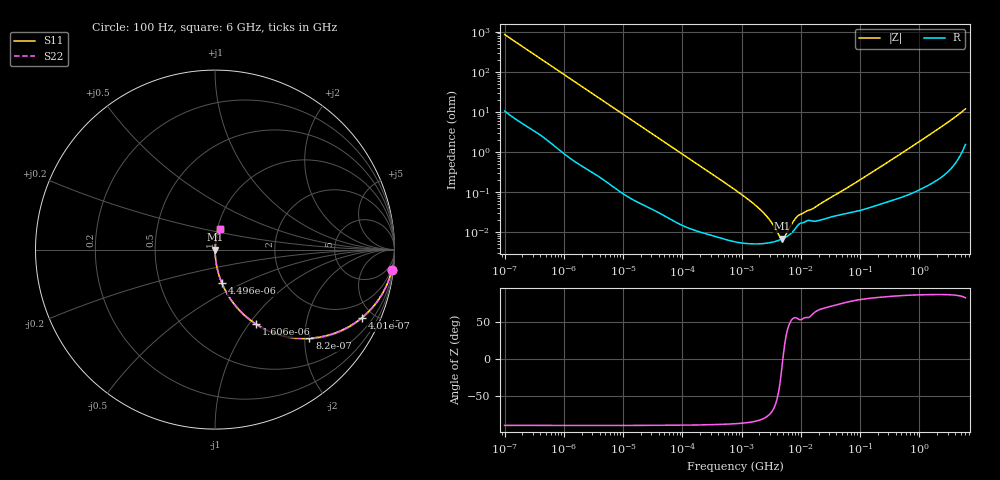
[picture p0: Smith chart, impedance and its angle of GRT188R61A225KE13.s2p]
!Murata Part Number: GRT188R61A225KE13
!These Parameters are Measured in Series Mode Connection
!Data Generated on Jun 19, 2026
!  o--ll--o
!Port1  Port2
!  o------o
!Operation Temp=25[degC], DC Bias Voltage=0[V]
!Freq. Start=100[Hz] Stop=6[GHz] 401[Steps]
# Hz S RI R 50
!Freq.(Hz) S11(Real) S11(Imag) S21(Real) S21(Imag) S12(Real) S12(Imag) S22(Real) S22(Imag)
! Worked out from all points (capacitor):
!   401 points, 100 Hz to 6 GHz, reference 50 ohm
!   read as one part in series: C = 1.87 uF near 109 Hz
!   lowest |Z| = 6.86 mohm at 4.857 MHz (marker M1)
!   series resonance near 4.978 MHz, so ESL is about 550 pH
!   S11 on the Smith chart (normalised r, x): 100 Hz: 1, -17; 401 Hz: 1.05, -4.29; 820 Hz: 1.02, -2.11; 1.606 kHz: 1.01, -1.08; 4.496 kHz: 1.00, -0.39; 6 GHz: 1.03, +0.24
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100  0.985 -0.1157  0.015 0.1157  0.015 0.1157  0.985 -0.1157
224  0.9332 -0.2437  0.0668 0.2437  0.0668 0.2437  0.9332 -0.2437
401  0.8183 -0.3795  0.1817 0.3795  0.1817 0.3795  0.8183 -0.3795
820  0.5256 -0.4939  0.4744 0.4939  0.4744 0.4939  0.5256 -0.4939
1122  0.3742 -0.4788  0.6258 0.4788  0.6258 0.4788  0.3742 -0.4788
1606  0.2281 -0.4146  0.7719 0.4146  0.7719 0.4146  0.2281 -0.4146
2008  0.16 -0.3615  0.84 0.3615  0.84 0.3615  0.16 -0.3615
4496  0.0382 -0.1864  0.9618 0.1864  0.9618 0.1864  0.0382 -0.1864
11514  0.00657 -0.0757  0.9934 0.0757  0.9934 0.0757  0.00657 -0.0757
40335  0.000786 -0.0219  0.9992 0.0219  0.9992 0.0219  0.000786 -0.0219
774597  5.91e-05 -0.00114  0.9999 0.00114  0.9999 0.00114  5.91e-05 -0.00114
2169299  5.19e-05 -0.00034  0.9999 0.00034  0.9999 0.00034  5.19e-05 -0.00034
2837864  5.42e-05 -0.000216  0.9999 0.000216  0.9999 0.000216  5.42e-05 -0.000216
4060267  6.14e-05 -7.49e-05  0.9999 7.49e-05  0.9999 7.49e-05  6.14e-05 -7.49e-05
4856642  6.8e-05 -8.9e-06  0.9999 8.9e-06  0.9999 8.9e-06  6.8e-05 -8.9e-06
5809218  7.82e-05 5.68e-05  0.9999 -5.68e-05  0.9999 -5.68e-05  7.82e-05 5.68e-05
7947587  0.000119 0.000175  0.9999 -0.000175  0.9999 -0.000175  0.000119 0.000175
9090158  0.000154 0.000211  0.9998 -0.000211  0.9998 -0.000211  0.000154 0.000211
1.555665e7  0.00019 0.000328  0.9998 -0.000328  0.9998 -0.000328  0.00019 0.000328
3.124326e8  0.000626 0.00587  0.9994 -0.00587  0.9994 -0.00587  0.000626 0.00587
1.95892e9  0.00318 0.0351  0.9968 -0.0351  0.9968 -0.0351  0.00318 0.0351
6e9  0.0283 0.1129  0.9717 -0.1129  0.9717 -0.1129  0.0283 0.1129
